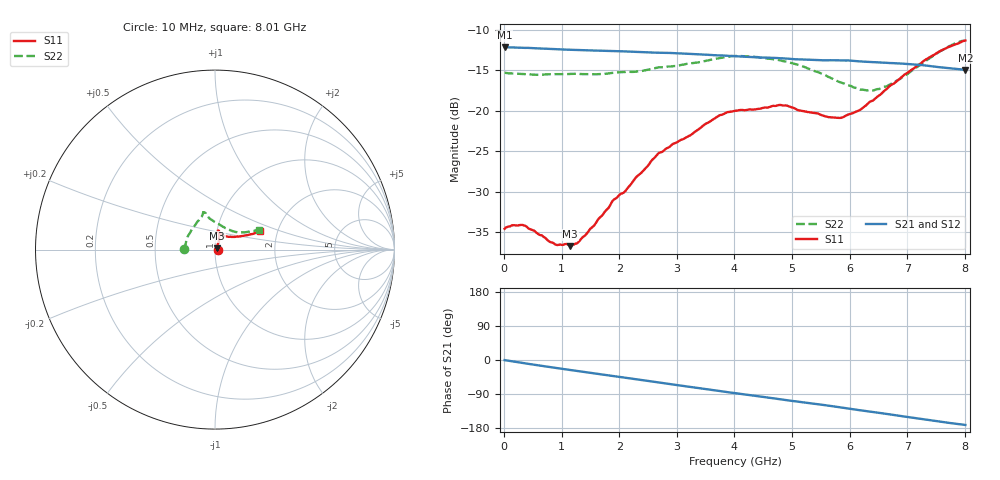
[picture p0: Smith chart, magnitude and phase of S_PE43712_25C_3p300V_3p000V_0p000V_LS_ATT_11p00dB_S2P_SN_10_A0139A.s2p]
! DEVICE ID: PE43712
! File Path: z:\PE43713\PE43713_CHAR_NOM_04292014\AMB\3p300\LS_ATT_11p00dB\PE43713_AMB_3p300V_3p000V_0p000V_LS_ATT_11p00dB_S2P_SN_10_A0139A.s2p
! Serial: 10
! Lot: A0139A
! Temp: 25C
! VDD: 3.300
! VSS: 0.000
! Control_Hi: 3.000
! Control_Lo: 0.000
! Attenuation Step: 11.00dB
! Port 1: RF1
! Port 2: RF2
! ThroughPath:1-2
! IDD: 0.0001470054
! ISS: -9.22e-008
#  Hz  S  RI  R  50
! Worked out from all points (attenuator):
!   801 points, 10 MHz to 8.01 GHz, reference 50 ohm
!   highest |S21| = -12.18 dB at 10 MHz (marker M1); lowest = -15.0 dB at 8.01 GHz (marker M2)
!   lowest |S11| = -36.7 dB at 1.15 GHz (marker M3), VSWR 1.03, Z = 51.2 + j0.845 ohm
!   |S11| at or under -10 dB: start of sweep to end of sweep
!   |S22| runs from -17.5 to -11.4 dB; largest |S21 - S12| = 0.00089
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1e7  0.0186 0.000272  0.2461 -0.00126  0.2462 -0.00126  -0.1713 0.00106
3.4e8  0.0195 -2.86e-05  0.2413 -0.035  0.2413 -0.0344  -0.1668 0.0205
8.9e8  0.0143 0.00411  0.2242 -0.0849  0.2243 -0.0849  -0.1596 0.0518
1.15e9  0.012 0.00825  0.2127 -0.1053  0.2128 -0.1056  -0.1545 0.0671
1.26e9  0.0118 0.00944  0.2076 -0.1136  0.2077 -0.1137  -0.1523 0.0726
1.35e9  0.012 0.0111  0.2033 -0.1204  0.2032 -0.1204  -0.1493 0.0772
1.57e9  0.0121 0.0155  0.1915 -0.1359  0.1915 -0.1359  -0.1412 0.0901
1.9e9  0.0136 0.0245  0.172 -0.1572  0.172 -0.1571  -0.1312 0.1099
2.11e9  0.0145 0.0285  0.1584 -0.1694  0.1584 -0.1693  -0.1248 0.12
2.68e9  0.0227 0.0495  0.1169 -0.1954  0.1168 -0.1954  -0.0968 0.1575
3.72e9  0.023 0.0895  0.0331 -0.2167  0.0329 -0.2167  -0.068 0.1989
4.01e9  0.0213 0.0974  0.00972 -0.2166  0.00968 -0.2166  -0.0662 0.207
4.79e9  0.0186 0.1068  -0.0492 -0.2047  -0.0492 -0.2049  -0.0503 0.198
5.35e9  0.0291 0.0926  -0.0864 -0.1867  -0.0864 -0.1867  -0.0323 0.1754
5.64e9  0.0398 0.0819  -0.104 -0.1761  -0.104 -0.1762  -0.0109 0.1607
5.87e9  0.0501 0.0754  -0.119 -0.1658  -0.1188 -0.1659  0.00955 0.148
6.17e9  0.0701 0.0718  -0.1356 -0.1487  -0.1354 -0.1489  0.0415 0.1287
6.31e9  0.0838 0.071  -0.142 -0.1409  -0.1416 -0.141  0.0583 0.1197
6.68e9  0.1202 0.0717  -0.1575 -0.1179  -0.1572 -0.118  0.1021 0.1011
7.36e9  0.193 0.0842  -0.1756 -0.0695  -0.1754 -0.0695  0.1818 0.0992
7.72e9  0.2283 0.0942  -0.1774 -0.0446  -0.1774 -0.0447  0.2248 0.1071
8.01e9  0.2495 0.1059  -0.1762 -0.0266  -0.1761 -0.0269  0.2465 0.1113
